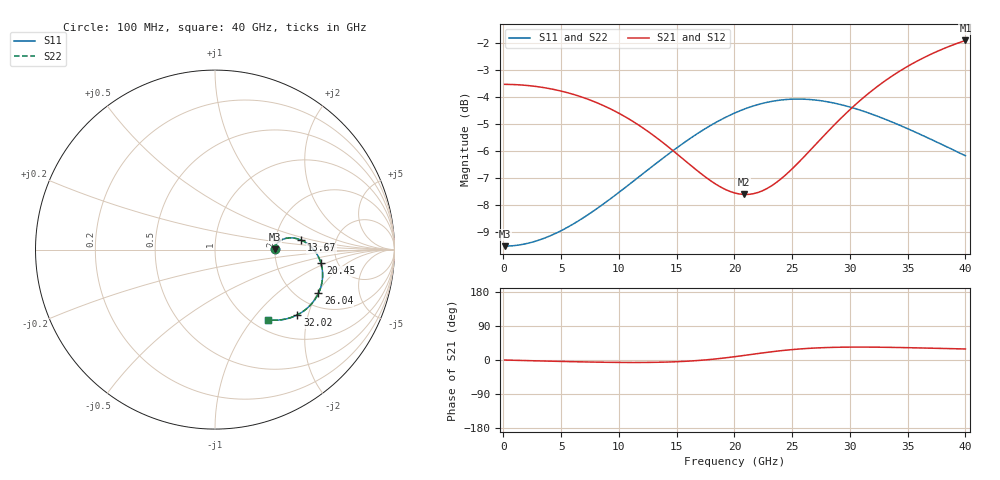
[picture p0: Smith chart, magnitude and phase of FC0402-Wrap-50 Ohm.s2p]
!Vishay Thin-Film
!FC Family
!Case Size 0402
!Assembly Style Full Wrap SMT
!10/21/2015
!thinfilm@vishay.com
# GHz S MA R 50
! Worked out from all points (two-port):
!   101 points, 100 MHz to 40 GHz, reference 50 ohm
!   highest |S21| = -1.89 dB at 40 GHz (marker M1); lowest = -7.6 dB at 20.85 GHz (marker M2)
!   |S21| within 3 dB of the highest: start of sweep to 11.16 GHz; 28.98 GHz to end of sweep
!   lowest |S11| = -9.5 dB at 100 MHz (marker M3), VSWR 2.00, Z = 100 + j0.204 ohm
!   |S11| at or under -10 dB: nowhere
!   |S22| runs from -9.5 to -4.1 dB; largest |S21 - S12| = 0
!   S11 on the Smith chart (normalised r, x): 100 MHz: 2.00, +0.00; 13.67 GHz: 2.81, +0.39; 20.45 GHz: 3.72, -0.87; 26.04 GHz: 2.55, -2.04; 32.02 GHz: 1.55, -1.71; 40 GHz: 1.17, -1.21
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0.1  0.3333 0.2  0.6667 -0.1  0.6667 -0.1  0.3333 0.2
3.292  0.3434 4.9  0.6585 -2.5  0.6585 -2.5  0.3434 4.9
6.883  0.3761 8.4  0.6303 -5.0  0.6303 -5.0  0.3761 8.4
10.474  0.4274 8.8  0.5813 -6.5  0.5813 -6.5  0.4274 8.8
12.07  0.4545 7.9  0.5533 -6.5  0.5533 -6.5  0.4545 7.9
13.666  0.4832 6.3  0.5223 -5.8  0.5223 -5.8  0.4832 6.3
15.262  0.5125 4.0  0.4901 -4.2  0.4901 -4.2  0.5125 4.0
16.858  0.5409 1.1  0.4593 -1.3  0.4593 -1.3  0.5409 1.1
18.454  0.5673 -2.4  0.4339 3.1  0.4339 3.1  0.5673 -2.4
20.05  0.59 -6.3  0.4185 8.8  0.4185 8.8  0.59 -6.3
20.449  0.5949 -7.3  0.4168 10.4  0.4168 10.4  0.5949 -7.3
20.848  0.5996 -8.3  0.416 12.1  0.416 12.1  0.5996 -8.3
22.045  0.6114 -11.6  0.4196 17.1  0.4196 17.1  0.6114 -11.6
23.242  0.6198 -15.0  0.432 21.8  0.432 21.8  0.6198 -15.0
24.439  0.6247 -18.4  0.4525 25.8  0.4525 25.8  0.6247 -18.4
26.035  0.6256 -22.9  0.489 29.9  0.489 29.9  0.6256 -22.9
26.833  0.6239 -25.2  0.5099 31.4  0.5099 31.4  0.6239 -25.2
29.626  0.608 -32.6  0.5878 33.9  0.5878 33.9  0.608 -32.6
32.02  0.5855 -38.4  0.6517 33.9  0.6517 33.9  0.5855 -38.4
33.616  0.5677 -41.8  0.6901 33.3  0.6901 33.3  0.5677 -41.8
36.409  0.5342 -47.2  0.7476 31.6  0.7476 31.6  0.5342 -47.2
40  0.491 -52.8  0.8046 29.1  0.8046 29.1  0.491 -52.8
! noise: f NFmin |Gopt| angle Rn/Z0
0.1  1.929e-15  1  -8.538e-07  1
4.489  3.857e-15  1  -1.479e-06  1.065
8.878  1.929e-15  1  -5.486e-15  1.284
13.27  2.893e-15  1  -8.538e-07  1.751
17.66  4.822e-15  1  -8.538e-07  2.488
22.05  4.822e-15  1  1.59e-14  2.557
26.43  9.643e-16  1  -8.538e-07  1.445
30.82  -1.446e-15  1  6.167e-15  0.6697
35.21  3.034e-08  1  3.656e-14  0.3316
40  0  1  1.069e-14  0.1724
